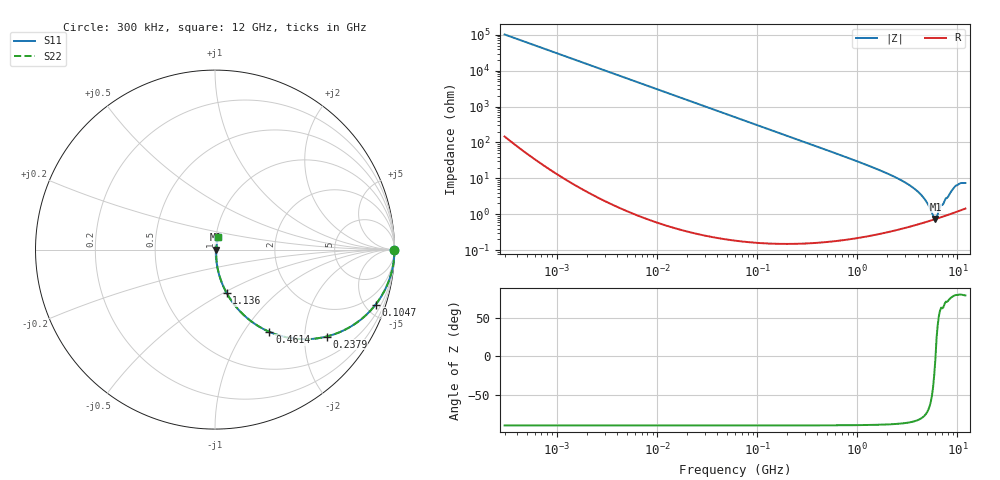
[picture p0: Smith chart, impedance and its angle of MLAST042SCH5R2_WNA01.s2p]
! MLAST042SCH5R2_WNA01  S-PARAMETER MODEL  ( General Type )
! Model Generated by TAIYO YUDEN Corporation (http://www.ty-top.com)
! Version 1.0
! TAIYO YUDEN Control No. 150820
! Copyright(c) 2015 TAIYO YUDEN CO.,LTD. All Rights Reserved.
! Product Description (link to TY-COMPAS)
! https://ds.yuden.co.jp/TYCOMPAS/or/detail?pn=MLAST042SCH5R2BWNA01&u=M
! Products Name : Multilayer Ceramic Capacitors
! Characteristics :
!  Capacitance : 5.2 pF , Rated Voltage : 25V , TCC : CH / C0H
!  Case Size : 0.4 x 0.2 / 0.016 x 0.008 [mm/inch] , Thickness : 0.2 / 0.008 [mm/inch]
!  (Conditions: Temperature = 25 degC , DC Bias Current/Voltage = 0A / 0V)
! External Node Assignments :
!  1  o---| |---o  2
! GND o---------o GND
! Frequency Range : 0.3MHz  -  12000MHz  [ 401 STEP ]
# MHz S RI R 50
! Freq[MHz].  S11 Real  S11 Imag  S21 Real  S21 Imag  S12 Real  S12 Imag  S22 Real  S22 Imag
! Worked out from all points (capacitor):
!   401 points, 300 kHz to 12 GHz, reference 50 ohm
!   read as one part in series: C = 5.2 pF near 316.3 kHz
!   lowest |Z| = 735 mohm at 6.026 GHz (marker M1)
!   series resonance near 6.042 GHz, so ESL is about 130 pH
!   S11 on the Smith chart (normalised r, x): 300 kHz: open; 104.7 MHz: 1.00, -5.84; 237.9 MHz: 1.00, -2.57; 461.4 MHz: 1.00, -1.32; 1.136 GHz: 1.00, -0.52; 12 GHz: 1.03, +0.15
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0.3  1 -0.000981  2.37e-06 0.000981  2.37e-06 0.000981  1 -0.000981
1.769972  1 -0.00579  3.52e-05 0.00579  3.52e-05 0.00579  1 -0.00579
10.44266  0.9988 -0.0341  0.00117 0.0341  0.00117 0.0341  0.9988 -0.0341
27.82928  0.9918 -0.0903  0.00824 0.0903  0.00824 0.0903  0.9918 -0.0903
60  0.9629 -0.1889  0.0371 0.1889  0.0371 0.1889  0.9629 -0.1889
104.6549  0.895 -0.3063  0.105 0.3063  0.105 0.3063  0.895 -0.3063
155.7172  0.7937 -0.4043  0.2063 0.4043  0.2063 0.4043  0.7937 -0.4043
237.9135  0.6221 -0.4843  0.3779 0.4843  0.3779 0.4843  0.6221 -0.4843
353.9943  0.4258 -0.4936  0.5742 0.4936  0.5742 0.4936  0.4258 -0.4936
461.3684  0.3032 -0.4584  0.6968 0.4584  0.6968 0.4584  0.3032 -0.4584
704.9044  0.1559 -0.3605  0.8441 0.3605  0.8441 0.3605  0.1559 -0.3605
1135.593  0.0651 -0.2423  0.9349 0.2423  0.9349 0.2423  0.0651 -0.2423
2088.533  0.0194 -0.1261  0.9806 0.1261  0.9806 0.1261  0.0194 -0.1261
3107.553  0.00941 -0.0715  0.9906 0.0715  0.9906 0.0715  0.00941 -0.0715
4050.141  0.00692 -0.0412  0.9931 0.0412  0.9931 0.0412  0.00692 -0.0412
4747.894  0.00653 -0.0245  0.9935 0.0245  0.9935 0.0245  0.00653 -0.0245
5715.274  0.00699 -0.00573  0.993 0.00573  0.993 0.00573  0.00699 -0.00573
6026.253  0.00729 -0.000369  0.9927 0.000369  0.9927 0.000369  0.00729 -0.000369
7064.448  0.00867 0.0158  0.9913 -0.0158  0.9913 -0.0158  0.00867 0.0158
9207.246  0.0136 0.052  0.9864 -0.052  0.9864 -0.052  0.0136 0.052
10236.47  0.0165 0.066  0.9835 -0.066  0.9835 -0.066  0.0165 0.066
12000  0.0193 0.0705  0.9807 -0.0705  0.9807 -0.0705  0.0193 0.0705
